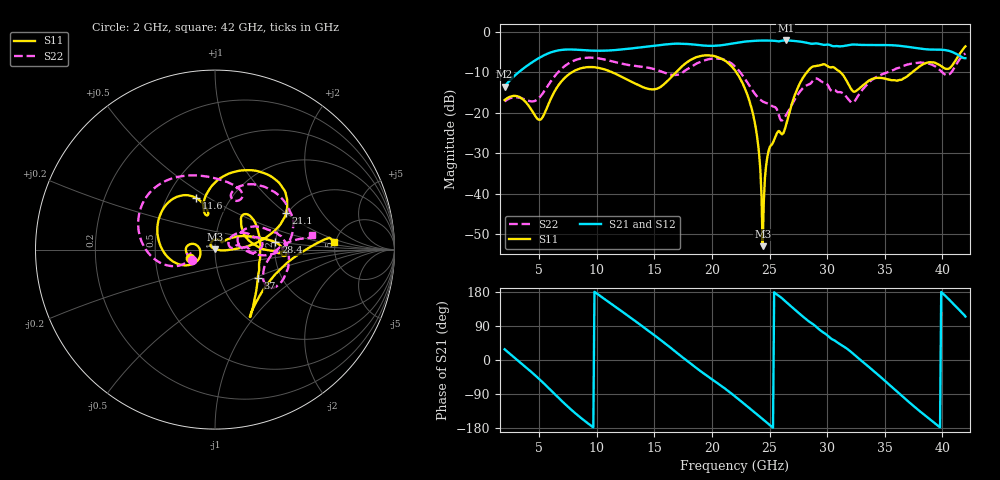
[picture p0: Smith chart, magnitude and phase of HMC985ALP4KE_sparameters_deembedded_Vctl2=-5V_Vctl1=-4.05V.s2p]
!s2p File: Measurements: S11, S21, S12, S22
# GHz S dB R 50.0
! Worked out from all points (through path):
!   401 points, 2 GHz to 42 GHz, reference 50 ohm
!   highest |S21| = -2.08 dB at 26.4 GHz (marker M1); lowest = -13.5 dB at 2 GHz (marker M2)
!   lowest |S11| = -52.9 dB at 24.4 GHz (marker M3), VSWR 1.00, Z = 50.1 + j0.193 ohm
!   |S11| at or under -10 dB: start of sweep to 7.815 GHz; 22.12 GHz to 28.23 GHz (6.101 GHz wide, 24.2 % of centre); 31.17 GHz to 37.36 GHz (6.192 GHz wide, 18.1 % of centre)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
!   |S22| runs from -21.9 to -5.3 dB; largest |S21 - S12| = 0.00074
!   S11 on the Smith chart (normalised r, x): 2 GHz: 0.76, -0.07; 11.6 GHz: 0.70, +0.44; 21.1 GHz: 1.97, +1.00; 28.4 GHz: 2.00, +0.19; 37 GHz: 1.52, -0.53; 42 GHz: 4.83, +0.78
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2  -16.80 -162.2  -13.46 28.3  -13.47 28.3  -17.15 -156.4
5  -21.70 -173.7  -6.40 -50.1  -6.40 -50.1  -16.25 -160.1
6.3  -14.87 -151.0  -4.78 -88.4  -4.78 -88.4  -11.08 -161.6
8.7  -8.91 150.1  -4.46 -154.6  -4.46 -154.6  -6.50 151.3
11.6  -10.29 110.1  -4.46 140.8  -4.46 140.9  -7.43 103.6
13.6  -13.12 100.9  -3.86 97.0  -3.86 97.0  -8.47 76.0
15.4  -13.81 105.5  -3.26 56.2  -3.26 56.2  -9.54 62.7
17.9  -7.33 79.8  -2.96 -3.8  -2.96 -3.8  -9.10 72.2
21.1  -7.04 27.2  -3.15 -74.7  -3.15 -74.7  -6.89 15.9
22  -9.48 16.6  -2.72 -96.0  -2.72 -95.9  -8.51 0.6
23.6  -20.74 0.0  -2.19 -135.7  -2.19 -135.7  -14.77 -3.5
24.4  -52.91 58.4  -2.11 -155.9  -2.10 -155.9  -17.15 7.7
25  -28.55 132.5  -2.13 -171.2  -2.13 -171.1  -17.82 11.0
26.4  -23.32 43.6  -2.08 154.1  -2.08 154.1  -20.68 32.9
28.4  -9.40 7.1  -2.77 102.1  -2.77 102.1  -12.98 18.2
28.7  -8.59 1.9  -2.90 96.0  -2.90 96.0  -12.23 16.5
30.7  -8.98 -3.3  -3.48 50.5  -3.48 50.5  -14.36 2.4
32.5  -14.59 34.1  -3.10 10.1  -3.11 10.1  -16.62 29.4
35.4  -11.75 18.5  -3.24 -65.3  -3.23 -65.2  -9.78 19.3
37  -10.83 -33.8  -3.66 -108.4  -3.66 -108.3  -8.03 4.8
39.8  -8.24 -56.5  -4.36 -177.9  -4.36 -177.9  -9.44 -34.5
42  -3.55 3.9  -6.46 114.6  -6.47 114.6  -5.28 8.6
